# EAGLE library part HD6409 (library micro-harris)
MICROCONTROLLER/MEMORY DEVICE
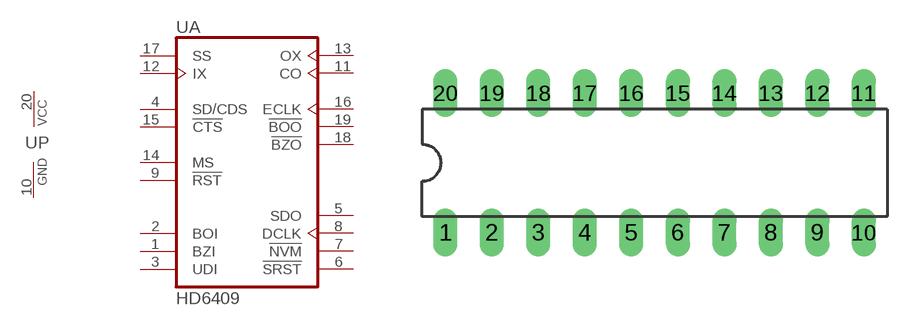
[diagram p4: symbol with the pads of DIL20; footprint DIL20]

Designator prefix U; gates A=HD6409 P=PWRN

## HD6409 (OC_FARNELL: unknown; OC_NEWARK: unknown)  [DIL20]
1  A:BZI  in
2  A:BOI  in
3  A:UDI  in
4  A:SD/CDS
5  A:SDO  out
6  A:!SRST  out
7  A:!NVM  out
8  A:DCLK  out
9  A:!RST  in
10  P:GND  pwr
11  A:CO  out
12  A:IX  in
13  A:OX  out
14  A:MS  in
15  A:!CTS  in
16  A:ECLK  out
17  A:SS  in
18  A:!BZO  out
19  A:!BOO  out
20  P:VCC  pwr

## Footprint DIL20 (pad centres in mm)
Dual In Line Package
drill 0.813 long: 1 -11.43,-3.81; 2 -8.89,-3.81; 3 -6.35,-3.81; 4 -3.81,-3.81; 5 -1.27,-3.81; 6 1.27,-3.81; 7 3.81,-3.81; 8 6.35,-3.81; 9 8.89,-3.81; 10 11.43,-3.81; 11 11.43,3.81; 12 8.89,3.81; 13 6.35,3.81; 14 3.81,3.81; 15 1.27,3.81; 16 -1.27,3.81; 17 -3.81,3.81; 18 -6.35,3.81; 19 -8.89,3.81; 20 -11.43,3.81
